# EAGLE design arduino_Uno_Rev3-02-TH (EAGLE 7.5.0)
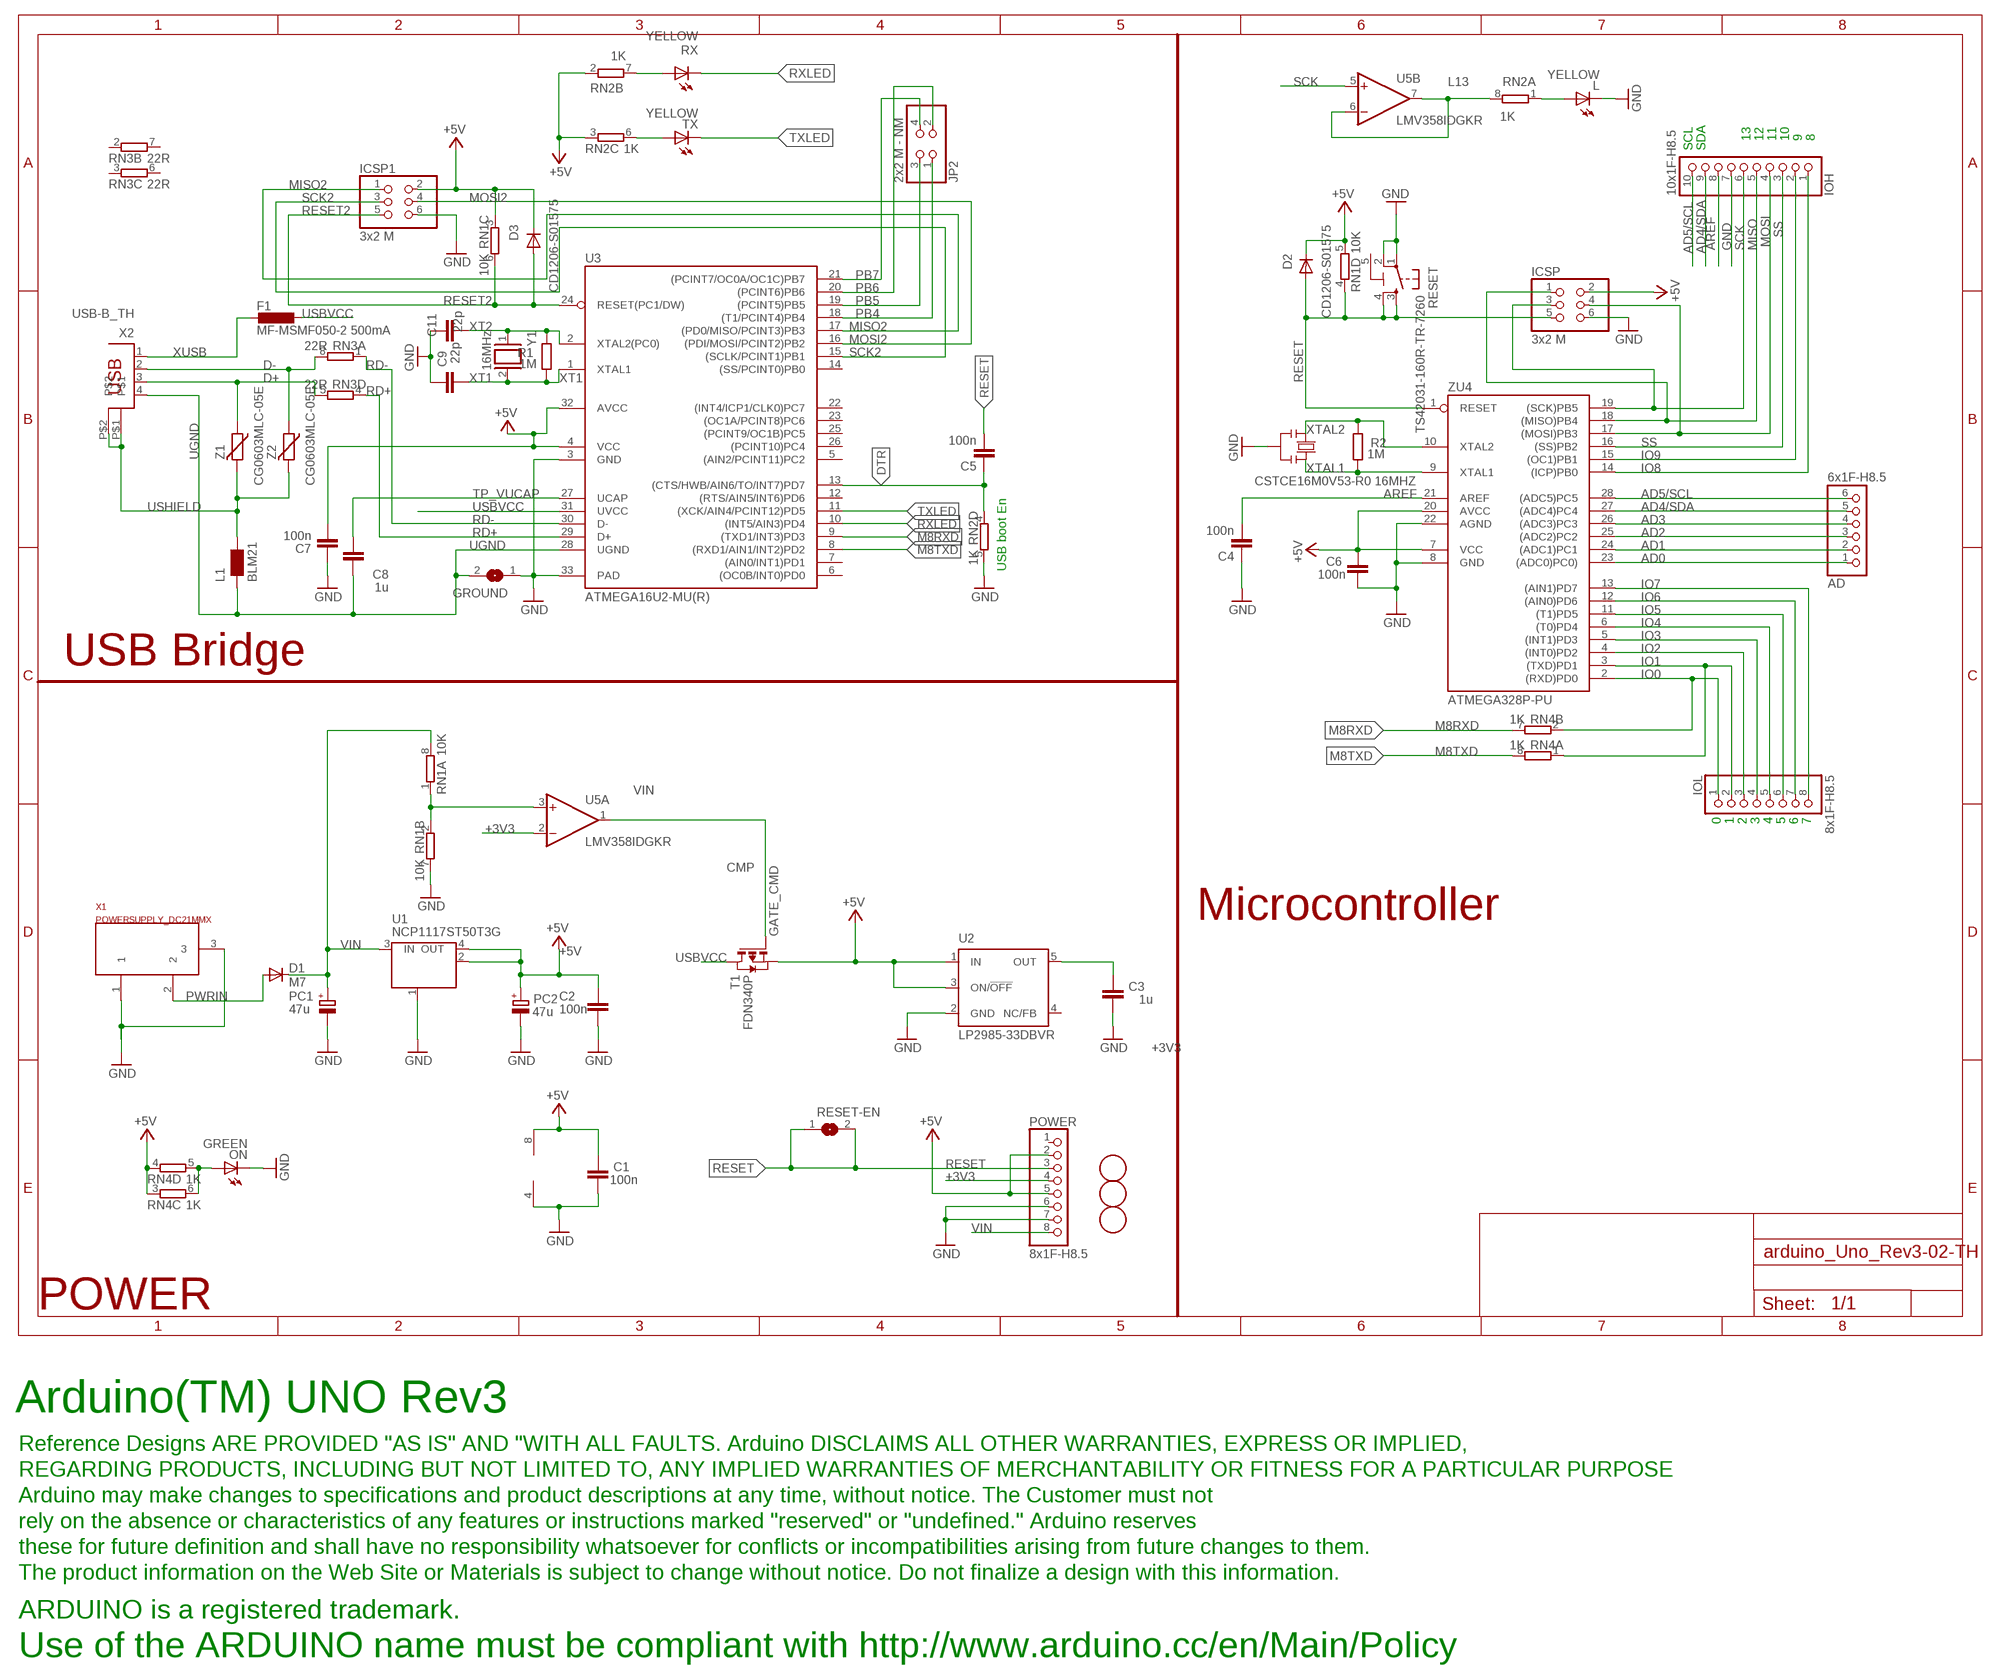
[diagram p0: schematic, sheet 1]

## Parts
AD  6x1F-H8.5  PINHD-1X6  [1X06]
C1  100n  C-EU0603-RND  [C0603-ROUND]
C2  100n  C-EU0603-RND  [C0603-ROUND]
C3  1u  C-EU0603-RND  [C0603-ROUND]
C4  100n  C-EU0603-RND  [C0603-ROUND]
C5  100n  C-EU0603-RND  [C0603-ROUND]
C6  100n  C-EU0603-RND  [C0603-ROUND]
C7  100n  C-EU0603-RND  [C0603-ROUND]
C8  1u  C-EU0603-RND  [C0603-ROUND]
C9  22p  C-EU0603-RND  [C0603-ROUND]
C11  22p  C-EU0603-RND  [C0603-ROUND]
D1  M7  DIODE-SMB  [SMB]
D2  CD1206-S01575  DIODE-MINIMELF  [MINIMELF]
D3  CD1206-S01575  DIODE-MINIMELF  [MINIMELF]
F1  MF-MSMF050-2 500mA  L-EUL1812  [L1812]
FD1  FIDUCIALMOUNT  [FIDUCIA-MOUNT]
FD2  FIDUCIALMOUNT  [FIDUCIA-MOUNT]
FD3  FIDUCIALMOUNT  [FIDUCIA-MOUNT]
GROUND  SJ  [SJ]
ICSP  3x2 M  PINHD-2X3  [2X03]
ICSP1  3x2 M  PINHD-2X3  [2X03]
IOH  10x1F-H8.5  PINHD-1X10_ARD  [1X10]
IOL  8x1F-H8.5  PINHD-1X8  [1X08]
JP2  2x2 M - NM  PINHD-2X2  [2X02]
L  YELLOW  LEDCHIP-LED0805  [CHIP-LED0805]
L1  BLM21  WE-CBF_0805  [0805]
ON  GREEN  LEDCHIP-LED0805  [CHIP-LED0805]
PC1  47u  CPOL-EUD  [PANASONIC_D]
PC2  47u  CPOL-EUD  [PANASONIC_D]
POWER  8x1F-H8.5  PINHD-1X8  [1X08]
R1  1M  R-EU_R0603  [R0603-ROUND]
R2  1M  R-EU_R0603  [R0603-ROUND]
RESET  TS42031-160R-TR-7260  TS42  [TS42]
RESET-EN  SJ  [SJ]
RN1  10K  4R-NCAY16  [CAY16]
RN2  1K  4R-NCAY16  [CAY16]
RN3  22R  4R-NCAY16  [CAY16]
RN4  1K  4R-NCAY16  [CAY16]
RX  YELLOW  LEDCHIP-LED0805  [CHIP-LED0805]
T1  FDN340P  PMOSSOT23  [SOT-23]
TX  YELLOW  LEDCHIP-LED0805  [CHIP-LED0805]
U1  NCP1117ST50T3G  MC33269ST-3.3T3  [SOT223]
U2  LP2985-33DBVR  LP2985-XXDBVR33  [SOT23-DBV]
U3  ATMEGA16U2-MU(R)  ATMEGA16U2-MU  [MLF32]
U5  LMV358IDGKR  LMV358MMX  [MSOP08]
U$1  DISCLAIMER  [DISCLAIMER]
X1  POWERSUPPLY_DC21MMX  [POWERSUPPLY_DC-21MM]
X2  USB-B_TH  PN61729  [PN61729]
Y1  16MHz  XTAL/S  [QS]
Y2  CSTCE16M0V53-R0 16MHZ  RESONATORMU  [RESONATOR]
Z1  CG0603MLC-05E  VARISTORCN0603  [CT/CN0603]
Z2  CG0603MLC-05E  VARISTORCN0603  [CT/CN0603]
ZU4  ATMEGA328P-PU  [DIL28-3]

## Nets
+3V3: C3.2 POWER.4 U2.5(OUT) U5.2(A:-IN)
+5V [usbvcc]: C1.2 C2.2 C6.2 C7.1 D2.C D3.C ICSP1.2 ICSP.2 PC2.+ POWER.2 POWER.5 RN1.3 RN1.5 RN2.2 RN2.3 RN4.3 RN4.4 T1.2(S) U1.2(OUT) U1.4(OUT) U2.1(IN) U2.3(ON/!OFF) U3.4(VCC) U3.32(AVCC) U5.8(P:V+) ZU4.7(VCC) ZU4.20(AVCC)
AD0: AD.1 ZU4.23((ADC0)PC0))
AD1: AD.2 ZU4.24((ADC1)PC1)
AD2: AD.3 ZU4.25((ADC2)PC2)
AD3: AD.4 ZU4.26((ADC3)PC3)
AD4/SDA: AD.5 IOH.9 ZU4.27((ADC4)PC4)
AD5/SCL: AD.6 IOH.10 ZU4.28((ADC5)PC5)
AREF [aref]: C4.2 IOH.8 ZU4.21(AREF)
CMP: RN1.1 RN1.2 U5.3(A:+IN)
D+: RN3.5 X2.3 Z1.1
D-: RN3.8 X2.2 Z2.1
DTR: C5.1 RN2.4 U3.13((CTS/HWB/AIN6/TO/INT7)PD7)
GATE_CMD: T1.3(G) U5.1(A:OUT)
GND [gnd]: C1.1 C2.1 C3.1 C4.1 C6.1 C7.2 C9.2 C11.2 GROUND.1 ICSP1.6 ICSP.6 IOH.7 L.C ON.C PC1.- PC2.- POWER.6 POWER.7 RESET.1 RESET.2 RN1.7 RN2.5 U1.1(GND/ADJ) U2.2(GND) U3.3(GND) U3.33(PAD) U5.4(P:V-) X1.1 X1.3 Y2.2 ZU4.8(GND) ZU4.22(AGND)
IO0: IOL.1 RN4.2 ZU4.2((RXD)PD0)
IO1: IOL.2 RN4.1 ZU4.3((TXD)PD1)
IO2: IOL.3 ZU4.4((INT0)PD2)
IO3: IOL.4 ZU4.5((INT1)PD3)
IO4: IOL.5 ZU4.6((T0)PD4)
IO5: IOL.6 ZU4.11((T1)PD5)
IO6: IOL.7 ZU4.12((AIN0)PD6)
IO7: IOL.8 ZU4.13((AIN1)PD7)
IO8: IOH.1 ZU4.14((ICP)PB0)
IO9: IOH.2 ZU4.15((OC1)PB1)
L13: RN2.8 U5.6(B:-IN) U5.7(B:OUT)
M8RXD: RN4.7 U3.9((TXD1/INT3)PD3)
M8TXD: RN4.8 U3.8((RXD1/AIN1/INT2)PD2)
MISO: ICSP.1 IOH.5 ZU4.18((MISO)PB4)
MISO2: ICSP1.1 U3.17((PD0/MISO/PCINT3)PB3)
MOSI: ICSP.4 IOH.4 ZU4.17((MOSI)PB3)
MOSI2: ICSP1.4 U3.16((PDI/MOSI/PCINT2)PB2)
N$1: L.A RN2.1
N$3: ON.A RN4.5 RN4.6
N$35: RN2.7 RX.A
N$36: RN2.6 TX.A
PB4: JP2.1 U3.18((T1/PCINT4)PB4)
PB5: JP2.3 U3.19((PCINT5)PB5)
PB6: JP2.2 U3.20((PCINT6)PB6)
PB7: JP2.4 U3.21((PCINT7/OC0A/OC1C)PB7)
PWRIN [power]: D1.A X1.2
RD+: RN3.4 U3.29(D+)
RD-: RN3.1 U3.30(D-)
RESET: C5.2 D2.A ICSP.5 POWER.3 RESET-EN.1 RESET-EN.2 RESET.3 RESET.4 RN1.4 ZU4.1(RESET)
RESET2: D3.A ICSP1.5 RN1.6 U3.24(RESET(PC1/DW))
RXLED: RX.C U3.10((INT5/AIN3)PD4)
SCK: ICSP.3 IOH.6 U5.5(B:+IN) ZU4.19((SCK)PB5)
SCK2: ICSP1.3 U3.15((SCLK/PCINT1)PB1)
SS: IOH.3 ZU4.16((SS)PB2)
TP_VUCAP: C8.1 U3.27(UCAP)
TXLED: TX.C U3.11((XCK/AIN4/PCINT12)PD5)
UGND [gnd]: C8.2 GROUND.2 L1.1 U3.28(UGND) X2.4
USBVCC [usbvcc]: F1.1 T1.1(D) U3.31(UVCC)
USHIELD [gnd]: L1.2 X2.P$1 X2.P$2 Z1.2 Z2.2
VIN [power]: D1.C PC1.+ POWER.8 RN1.8 U1.3(IN)
XT1: C9.1 R1.1 U3.1(XTAL1) Y1.2
XT2: C11.1 R1.2 U3.2(XTAL2(PC0)) Y1.1
XTAL1: R2.1 Y2.3 ZU4.9(XTAL1)
XTAL2: R2.2 Y2.1 ZU4.10(XTAL2)
XUSB [usbvcc]: F1.2 X2.1
Unconnected: POWER.1 RN3.2 RN3.3 RN3.6 RN3.7 U2.4(NC/FB) U3.5((AIN2/PCINT11)PC2) U3.6((OC0B/INT0)PD0) U3.7((AIN0/INT1)PD1) U3.12((RTS/AIN5/INT6)PD6) U3.14((SS/PCINT0)PB0) U3.22((INT4/ICP1/CLK0)PC7) U3.23((OC1A/PCINT8)PC6) U3.25((PCINT9/OC1B)PC5) U3.26((PCINT10)PC4)

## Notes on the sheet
- 13 | 12 | 11 | 10 | 9 | 8
- SCL | SDA
- USB boot En
- USB Bridge
- 0 | 1 | 2 | 3 | 4 | 5 | 6 | 7
- Microcontroller
- POWER
- Arduino(TM) UNO Rev3
- Use of the ARDUINO name must be compliant with http://www.arduino.cc/en/Main/Policy

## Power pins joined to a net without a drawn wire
5-GND: RESET.5(5-GND)

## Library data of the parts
AD = SmartPrj:PINHD-1X6: PIN HEADER
C1-C9 C11 = SmartPrj:C-EU: CAPACITOR, European symbol
D1-D3 = diode:DIODE-: DIODE
F1 = rcl:L-EU: INDUCTOR, European symbol
FD1-FD3 = SmartPrj:FIDUCIALMOUNT
GROUND RESET-EN = jumper:SJ: SMD solder JUMPER
ICSP ICSP1 = SmartPrj:PINHD-2X3: PIN HEADER
IOH = SmartPrj:PINHD-1X10_ARD: PIN HEADER
IOL POWER = SmartPrj:PINHD-1X8: PIN HEADER
JP2 = SmartPrj:PINHD-2X2: PIN HEADER
L ON RX TX = led:LED: LED
L1 = wuerth-elektronik:WE-CBF: SMD EMI Suppression Ferrite Beads
PC1 PC2 = rcl:CPOL-EU: POLARIZED CAPACITOR, European symbol
R1 R2 = SmartPrj:R-EU_: RESISTOR, European symbol
RESET = SmartPrj:TS42: TS42 Dongnan Electronics Tact switch VDC 12V - 50mA
RN1-RN4 = resistor-dil:4R-N: Array Chip Resistor Source: RS Component / Phycomp
T1 = zetex:PMOSSOT23: MOS FET
U1 = linear:MC33269ST*: Adjustable Output Low Dropout Voltage Regulator 800 mA Source: http://www.onsemi.com/pub/Collateral/MC33269-D.PDF
U2 = SmartPrj:LP2985-XXDBVR: ULTRALOW-POWER 50-mA LOW-DROPOUT LINEAR REGULATORS 50-mA Low-Dropout Regulator Source: http://focus.ti.com/lit/ds/symlink/tps77001.pdf
U3 = SmartPrj:ATMEGA16U2-
U5 = linear:LMV358?*: Dual General Purpose, Low Voltage, Rail-to-Rail Output Operational Amplifiers Source: http://www.national.com/mpf/LM/LMV321.html http://www.national.com/dt/lmv_qual.pdf
U$1 = SmartPrj:DISCLAIMER
X1 = SmartPrj:POWERSUPPLY_DC21MM
X2 = SmartPrj:PN61729: BERG USB connector
Y1 = SmartPrj:XTAL/S: CRYSTAL
Y2 = SmartPrj:RESONATOR
Z1 Z2 = varistor:VARISTOR: VARISTOR
ZU4 = SmartPrj:ATMEGA328P-: MICROCONTROLLER 4 Kbytes FLASH 128 bytes SRAM 256 bytes EEPROM UART 6-channel 10 bit ADC

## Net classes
0 default: width 0.254 mm, clearance 0.254 mm
1 power: width 0.61 mm, drill 0.61 mm, clearance 0.254 mm
2 gnd: width 0.305 mm, drill 0.559 mm, clearance 0.254 mm
3 usbvcc: width 0.508 mm, drill 0.61 mm, clearance 0.254 mm
4 aref: width 0.406 mm, drill 0.61 mm, clearance 0.254 mm

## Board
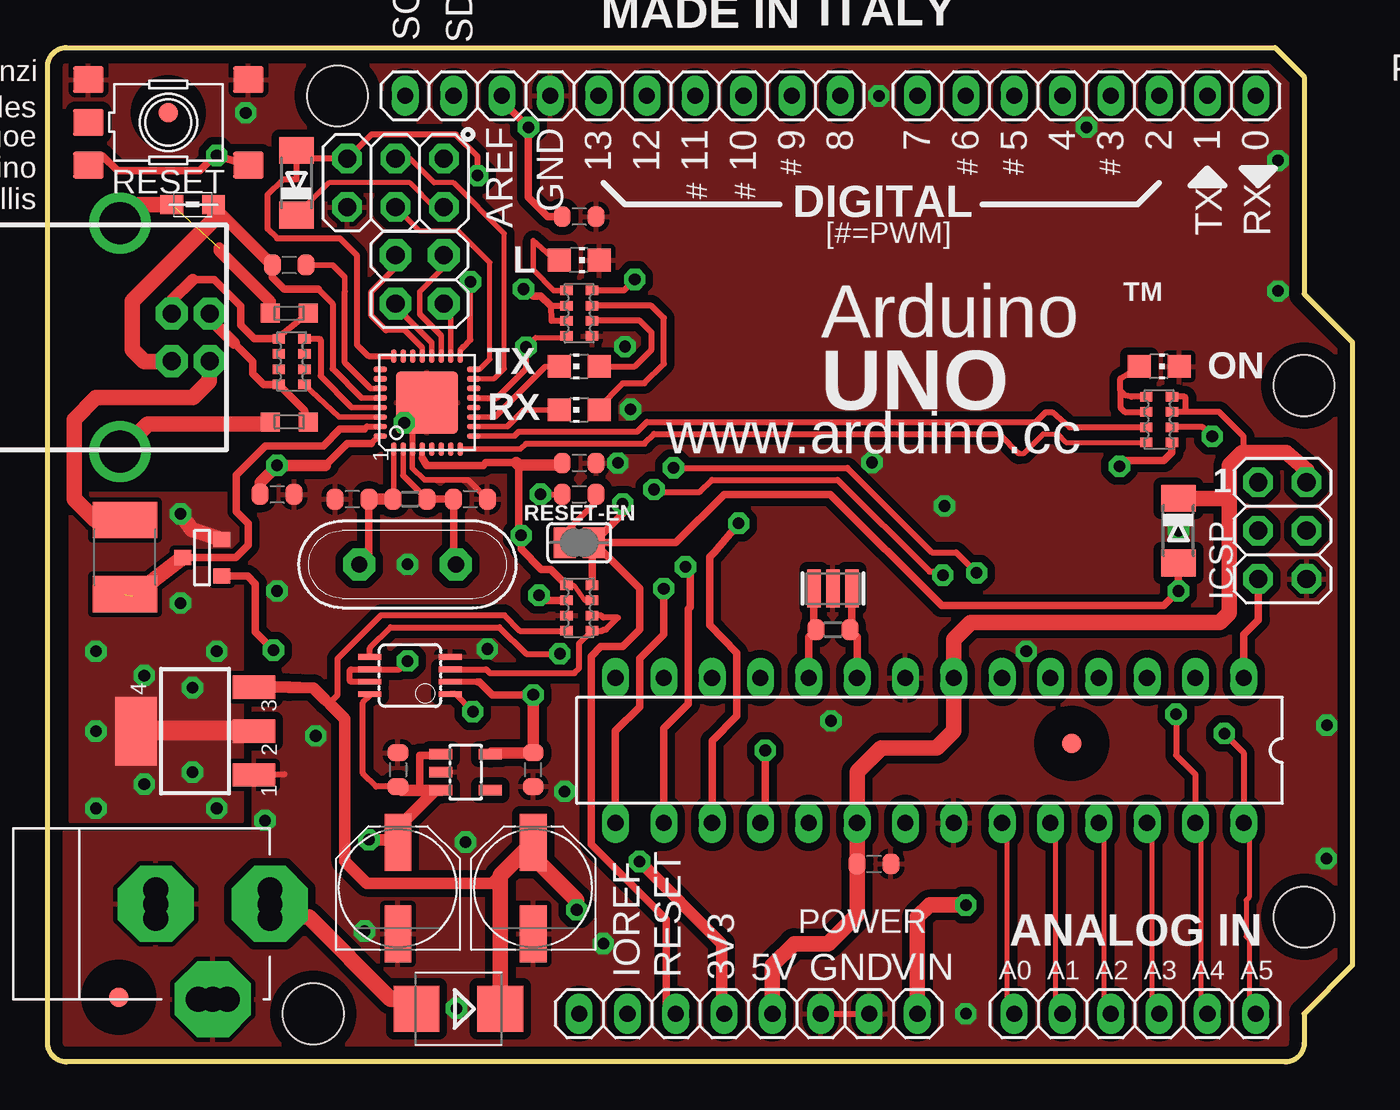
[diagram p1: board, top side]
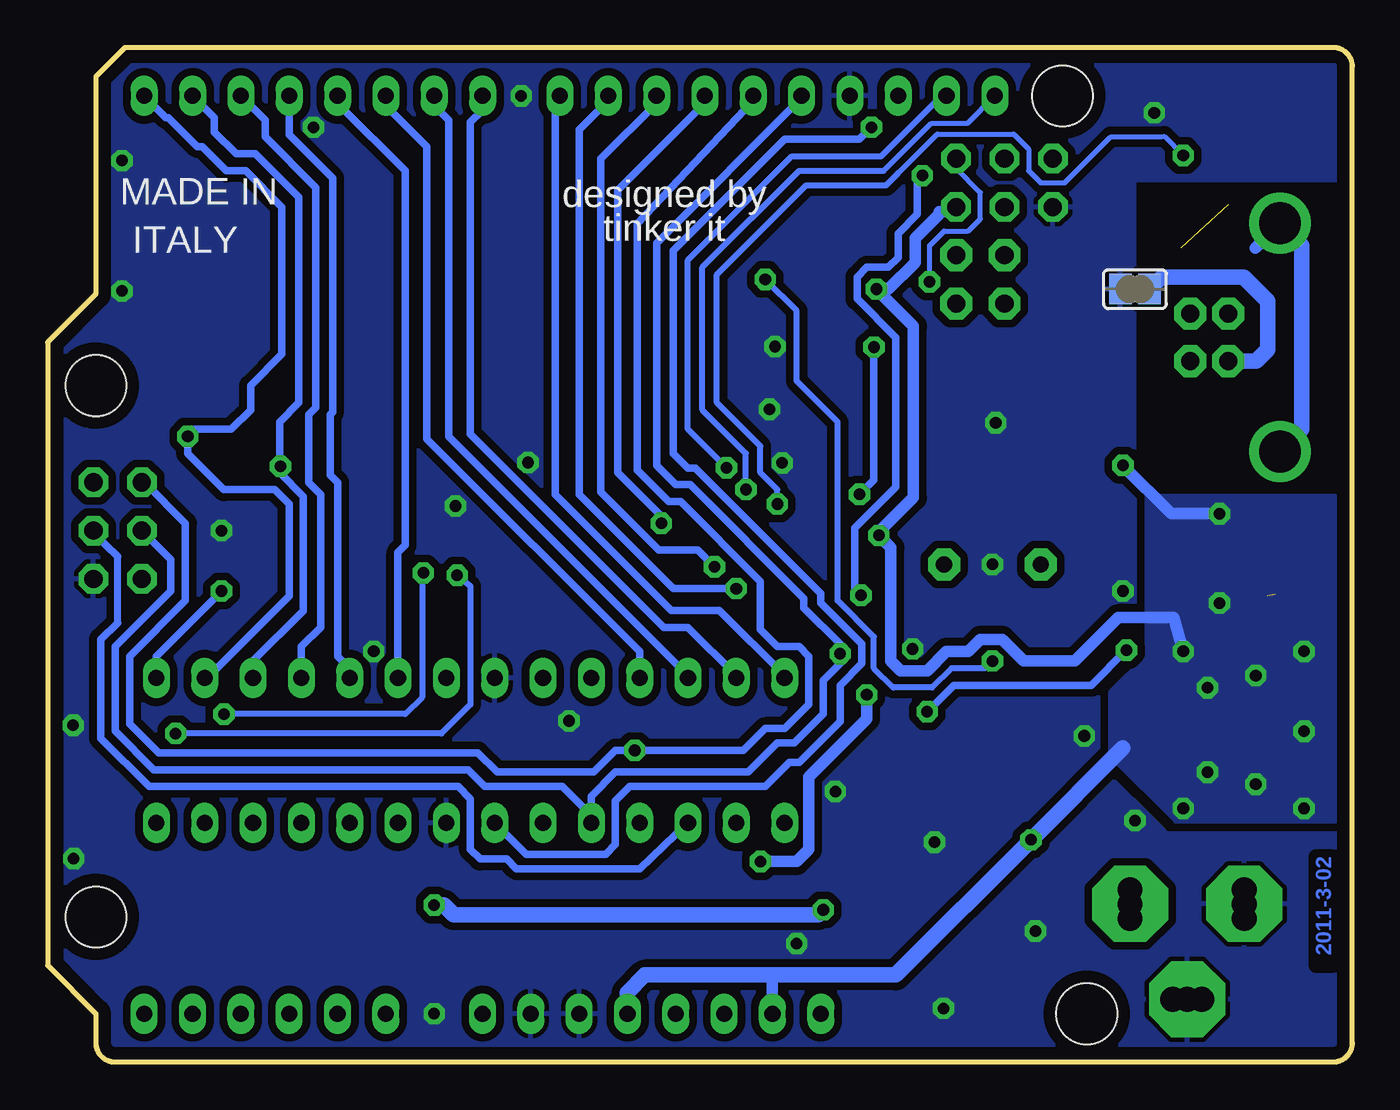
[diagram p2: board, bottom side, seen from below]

Size 68.58 x 53.34 mm. Coordinates in mm from the lower left corner, seen from the top.
Outline: 64.52,53.34 66.04,51.82 66.04,40.39 68.58,37.85 68.58,5.08 66.04,2.54 66.04,1 arc-90 65.04,0 1,0 arc-90 0,1 0,52.34 arc-90 1,53.34 64.52,53.34
Copper layers (1*16): Top 0.035mm / dielectric 1.5mm / Bottom 0.035mm
Design rules: minimum track width 10mil, minimum drill 22mil, track to track 10mil, track to pad 10mil, pad to pad 10mil, via to via 12mil, smd to smd 8mil, copper to edge 26mil, drill to drill 12mil, minimum pad ring 10mil, minimum via ring 10mil, stop-mask expansion 1mil, vias tented up to drill 30mil, thermal gap 10mil
Holes 3.2 mm at 66.04,35.56 66.04,7.62 15.24,50.8 13.97,2.54
vRestrict: area 22.9,44.1 to 24.6,49.1; area 25.4,45.5 to 27.1,49.1; area 28.4,45.3 to 29.6,48.8; area 31,45.3 to 32.1,48.8; area 33.5,45.3 to 34.7,48.8; area 36.1,45.3 to 37.2,48.8; area 38.7,47.2 to 39.9,48.8; area 40.3,45.1 to 47.6,46.9; area 60.3,44.2 to 61.7,46.7; area 62.9,44.2 to 64.3,46.7; area 61.3,35.8 to 64.8,37.2; area 0.6,21.8 to 2,30.1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

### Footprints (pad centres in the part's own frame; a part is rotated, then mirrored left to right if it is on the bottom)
1X06 = drill 0.85 pad 1.422 long: 1 -6.35,0; 2 -3.81,0; 3 -1.27,0; 4 1.27,0; 5 3.81,0; 6 6.35,0
C0603-ROUND = smd 0.898 x 1.1: 1 -0.889,0; 2 0.889,0
SMB = smd 2.4 x 2.4: A 2.2,0; C -2.2,0
MINIMELF = smd 1.4 x 1.8: A 1.7,0; C -1.7,0
L1812 = smd 1.9 x 3.4: 1 -1.95,0; 2 1.95,0
FIDUCIA-MOUNT = smd 1.016 x 1.016: P$1 0,0
SJ = smd 1.168 x 1.6: 1 -0.762,0; 2 0.762,0
2X03 = drill 0.95 pad 1.55 octagon: 1 -2.54,-1.27; 2 -2.54,1.27; 3 0,-1.27; 4 0,1.27; 5 2.54,-1.27; 6 2.54,1.27
1X10 = drill 0.85 pad 1.422 long: 1 -11.43,0; 2 -8.89,0; 3 -6.35,0; 4 -3.81,0; 5 -1.27,0; 6 1.27,0; 7 3.81,0; 8 6.35,0; 9 8.89,0; 10 11.43,0
1X08 = drill 0.85 pad 1.422 long: 1 -8.89,0; 2 -6.35,0; 3 -3.81,0; 4 -1.27,0; 5 1.27,0; 6 3.81,0; 7 6.35,0; 8 8.89,0
2X02 = drill 0.95 pad 1.676 octagon: 1 -1.27,-1.27; 2 -1.27,1.27; 3 1.27,-1.27; 4 1.27,1.27
CHIP-LED0805 = smd 1.2 x 1.2: A 0,-1.05; C 0,1.05
0805 = smd 1.2 x 1: 1 -1.1,0; 2 1.1,0
PANASONIC_D = smd 3 x 1.4: + 2.4,0; - -2.4,0
R0603-ROUND = smd 0.898 x 1.1: 1 -0.889,0; 2 0.889,0
TS42 = smd 1.6 x 1.4: 1 -4.2,2.25; 2 4.2,2.25; 3 -4.2,-2.25; 4 4.2,-2.25; 5 -4.2,0
CAY16 = smd 0.5 x 0.65: 1 -1.2,-0.675; 2 -0.4,-0.675; 3 0.4,-0.675; 4 1.2,-0.675; 5 1.2,0.675; 6 0.4,0.675; 7 -0.4,0.675; 8 -1.2,0.675
SOT-23 = smd 0.787 x 0.889: 1 0.025,-1.016; 2 -0.94,1.016; 3 0.991,1.016
SOT223 = smd 1.219 x 2.235: 1 -2.311,-3.099; 2 0,-3.099; 3 2.311,-3.099 | smd 3.6 x 2.2: 4 0,3.099
SOT23-DBV = smd 0.55 x 1.2: 1 -0.95,-1.3; 2 0,-1.3; 3 0.95,-1.3; 4 0.95,1.3; 5 -0.95,1.3
MLF32 = smd 0.7 x 0.28: 1 -2.45,1.75; 2 -2.45,1.25; 3 -2.45,0.75; 4 -2.45,0.25; 5 -2.45,-0.25; 6 -2.45,-0.75; 7 -2.45,-1.25; 8 -2.45,-1.75; 17 2.45,-1.75; 18 2.45,-1.25; 19 2.45,-0.75; 20 2.45,-0.25; 21 2.45,0.25; 22 2.45,0.75; 23 2.45,1.25; 24 2.45,1.75 | smd 0.28 x 0.7: 9 -1.75,-2.45; 10 -1.25,-2.45; 11 -0.75,-2.45; 12 -0.25,-2.45; 13 0.25,-2.45; 14 0.75,-2.45; 15 1.25,-2.45; 16 1.75,-2.45; 25 1.75,2.45; 26 1.25,2.45; 27 0.75,2.45; 28 0.25,2.45; 29 -0.25,2.45; 30 -0.75,2.45; 31 -1.25,2.45; 32 -1.75,2.45 | smd 3.254 x 3.254: 33 0,0
MSOP08 = smd 0.3 x 1.2: 1 -0.976,-2.113; 2 -0.326,-2.113; 3 0.324,-2.113; 4 0.974,-2.113; 5 0.974,2.112; 6 0.324,2.112; 7 -0.326,2.112; 8 -0.976,2.112
POWERSUPPLY_DC-21MM = drill 1.3 pad 4 octagon: 1 -5.08,-3.353; 2 -0.076,-6.35; 3 -0.076,-0.356 | drill 1.3: 4 -5.08,-4.115; 5 -5.08,-2.591; 6 -0.838,-0.356; 7 0.686,-0.356; 8 -0.838,-6.35; 9 0.686,-6.35
PN61729 = drill 0.95 pad 1.676 octagon: 1 1.25,4.71; 2 -1.25,4.71; 3 -1.25,2.71; 4 1.25,2.71 | drill 2.2: P$1 -6,0; P$2 6,0
QS = drill 0.85 pad 1.676 octagon: 1 -2.54,0; 2 2.54,0
RESONATOR = smd 0.7 x 2: 1 -1,0; 2 0,0; 3 1,0
CT/CN0603 = smd 1 x 1: 1 -1,0; 2 1,0
DIL28-3 = drill 0.85 pad 1.422 long: 1 -16.51,-3.81; 2 -13.97,-3.81; 3 -11.43,-3.81; 4 -8.89,-3.81; 5 -6.35,-3.81; 6 -3.81,-3.81; 7 -1.27,-3.81; 8 1.27,-3.81; 9 3.81,-3.81; 10 6.35,-3.81; 11 8.89,-3.81; 12 11.43,-3.81; 13 13.97,-3.81; 14 16.51,-3.81; 15 16.51,3.81; 16 13.97,3.81; 17 11.43,3.81; 18 8.89,3.81; 19 6.35,3.81; 20 3.81,3.81; 21 1.27,3.81; 22 -1.27,3.81; 23 -3.81,3.81; 24 -6.35,3.81; 25 -8.89,3.81; 26 -11.43,3.81; 27 -13.97,3.81; 28 -16.51,3.81

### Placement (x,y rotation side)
AD  57.15,2.54 0 top
C1  18.41,15.37 270 top
C2  12.06,29.84 180 top
C3  25.53,15.37 90 top
C4  27.94,44.45 180 top
C5  27.94,29.84 0 top
C6  43.43,10.41 180 top
C7  27.94,31.5 0 top
C8  12.7,41.91 180 top
C9  16,29.59 180 top
C11  22.23,29.59 0 top
D1  21.59,2.79 180 top
D2  59.44,27.94 270 top
D3  13.08,46.23 90 top
F1  4.06,26.54 90 top
FD1  6.35,49.91 0 top
FD2  53.84,16.74 0 top
FD3  3.73,3.41 0 top
GROUND  11.43,40.64 0 bottom
ICSP  64.9,27.94 270 top
ICSP1  18.29,46.23 180 top
IOH  30.23,50.8 180 top
IOL  54.61,50.8 180 top
JP2  19.56,41.15 90 top
L  27.94,42.16 270 top
L1  7.62,45.09 180 top
ON  58.42,36.58 270 top
PC1  25.53,9.14 90 top
PC2  18.41,9.14 90 top
POWER  36.83,2.54 0 top
R1  19.05,29.59 0 top
R2  41.27,22.73 180 top
RESET  6.35,49.4 0 top
RESET-EN  27.94,27.3 0 top
RN1  27.94,23.88 90 top
RN2  27.94,39.37 270 top
RN3  12.83,36.83 90 top
RN4  58.42,33.78 90 top
RX  27.94,34.29 90 top
T1  8.13,26.54 270 top
TX  27.94,36.58 90 top
U1  7.75,17.4 90 top
U2  21.97,15.24 270 top
U3  19.94,34.67 90 top
U5  19.05,20.32 90 top
U$1  not placed on the board
X1  5.33,8.38 90 top
X2  3.81,38.1 270 top
Y1  18.92,26.16 180 top
Y2  41.27,24.89 0 top
Z1  12.7,39.37 180 top
Z2  12.7,33.66 180 top
ZU4  46.35,16.38 180 top

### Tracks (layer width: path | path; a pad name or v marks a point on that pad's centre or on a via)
+3V3  (via drill 0.61)
  Top 0.305: 22.61,19.99 U5.2
  Top 0.406: 22.61,19.99 22.68,19.99 23.37,19.3 v25.53,19.3
  Top 0.61: v31.11,10.54 35.43,6.22 35.43,2.67 POWER.4 | U2.5 23.34,16.26 C3.2 v25.53,19.3
  Bottom 0.61: v31.11,10.54 29.21,10.54 28.57,11.18 28.57,14.99 25.53,18.03 v25.53,19.3
+5V  (via drill 0.61)
  Top 0.254: 27.32,25.02 RN1.5 27.65,25.08 28.23,24.28 RN1.3 | ICSP1.2 20.32,44.96 19.05,46.23 14.78,46.23 D3.C
  Top 0.305: 59.82,34.18 61.58,34.18 62.87,32.89 62.87,32.05 | 59.82,34.18 RN4.3 | RN4.4 59.76,34.98 59.82,34.92 59.82,34.18 | RN2.2 26.43,39.77 26.47,38.97 RN2.3 | 19.69,31.75 U3.4 | U3.32 17.43,32.92 17.02,32.51 | U5.8 16.98,19.3 16.57,18.9 16.57,15.18 17.27,14.48 C1.2
  Top 0.406: 42.55,10.16 42.35,10.35 | 26.43,39.77 25.93,40.28 25.53,40.26 v25.02,40.64 | RN1.5 26.43,25.91 25.96,25.91 24.89,26.97 v24.89,27.69 24.77,28.19 24.77,31.38 | 24.64,31.51 23.03,31.51 22.89,31.37 19.94,31.37 19.69,31.75 | 17.02,32.51 15.75,32.51 14.61,31.37 | U2.1 20.61,16.13 19.56,16.13 19.56,14.29
  Top 0.508: 11.02,17.42 U1.2 | ICSP.2 66.04,30.48
  Top 0.61: C6.2 42.58,10.88 42.55,11.43 | 24.64,31.51 24.77,31.38 26.94,31.38 C7.1 | 11.05,29.72 C2.2 11.18,30.48 v12.06,31.37 14.61,31.37 | v16.89,11.68 18.78,11.68 PC2.+ 18.41,12.32 20.39,14.29 U2.3 19.56,14.29 18.6,14.29 C1.2
  Top 0.813: 66.17,30.44 ICSP.2 66.17,31.11 65.1,32.05 62.87,32.05 62.79,32.05 62.1,31.37 62.1,29.46 | 62.1,29.46 62.1,23.62 61.59,23.11 48.51,23.11 47.62,22.23 ZU4.7 47.62,17.4 46.74,16.51 43.81,16.51 42.55,15.24 ZU4.20 42.55,11.43 C6.2 42.55,10.16 42.55,7.75 41.02,6.22 39.24,6.22 38.1,5.08 POWER.5 | T1.2 7.57,27.99 v6.99,28.83 | D2.C 61.93,29.64 62.1,29.46
  Top 1.016: U1.4 5.84,17.4 5.87,17.42 11.02,17.42
  Bottom 0.61: ICSP1.2 21.08,44.7 21.72,44.7 21.72,44.58 22.99,43.31 22.99,42.04 24.38,40.64 v25.02,40.64 23.07,38.69 23.07,29.68 24.89,27.85 v24.89,27.69 24.26,27.05 24.26,21.08 23.75,20.57 22.35,20.57 21.34,21.59 20.19,21.59 19.56,22.23 18.41,22.23 17.27,21.08 14.61,21.08 12.32,23.37 9.4,23.37 v8.89,21.59 | POWER.2 30.48,4.7 30.61,4.57 | v12.06,31.37 9.53,28.83 v6.99,28.83
  Bottom 0.813: POWER.5 38.12,3.63 37.19,4.57 30.61,4.57 24,4.57 v16.89,11.68 12.06,16.51
  other vias: 2.54,21.59 5.08,20.32 6.99,24.13 2.54,13.34 5.08,14.61 2.54,17.4 8.89,13.34 7.62,15.24 7.62,19.68
  pour Bottom (isolate 0.406, no thermals): 0.89,29.72 10.79,29.72 10.79,21.34 12.7,19.43 12.7,16.13 9.27,12.7 0.89,12.7
  pour Top (no thermals): 1.27,12.7 1.27,29.84 10.16,29.84 10.16,12.7
AD0
  Top 0.254: ZU4.23 50.44,12.17 50.44,3 AD.1
AD1
  Top 0.254: ZU4.24 52.98,12.17 52.98,3 AD.2
AD2
  Top 0.254: ZU4.25 55.52,12.17 55.52,3 AD.3
AD3
  Top 0.254: ZU4.26 58.06,12.17 58.06,3 AD.4
AD4/SDA  (via drill 0.61)
  Top 0.254: ZU4.27 60.6,12.17 60.6,3 AD.5
  Top 0.305: v32.89,31.24 42.04,31.24 46.48,26.8 47.75,26.8 v48.83,25.72 49.02,25.65 | v59.31,18.29 59.31,16.13 60.33,15.11 ZU4.27
  Bottom 0.305: IOH.9 21.59,50.8 24.77,47.62 29.46,47.62 34.92,42.16 34.92,33.27 v32.89,31.24 | v48.83,25.72 48.9,25.65 48.9,19.18 49.78,18.29 v59.31,18.29
AD5/SCL  (via drill 0.61)
  Top 0.254: ZU4.28 63.14,12.17 63.14,8.66 62.99,8.51 62.99,6.6 63.14,6.45 63.14,3 AD.6
  Top 0.305: v31.88,30.1 31.88,29.97 34.29,29.97 34.92,30.61 41.53,30.61 46.35,25.78 46.86,25.78 v47.05,25.59 | ZU4.28 62.87,16.26 v61.85,17.27
  Bottom 0.254: IOH.10 20.22,49.35 22.12,49.35 24.64,46.86
  Bottom 0.305: v61.85,17.27 47.88,17.27 46.35,18.8 46.35,25.02 v47.05,25.59 | v31.88,30.1 31.88,32 34.16,34.29 34.16,41.78 29.08,46.86 24.64,46.86
AREF  (via drill 0.61)
  Top 0.406: IOH.8 23.88,50.55 v25.27,49.15 25.27,45.47 26.29,44.45 C4.2
  Bottom 0.406: ZU4.21 43.43,10.92 39.24,10.92 38.73,11.43 38.73,13.72 37.97,14.48 30.86,14.48 29.59,15.75 29.08,15.75 26.92,17.91 26.92,19.81 25.78,20.95 25.78,21.97 27.94,24.13 27.94,24.64 34.54,31.24 34.92,31.24 35.69,32 35.69,42.67 29.84,48.51 25.91,48.51 v25.27,49.15
CMP
  Top 0.305: U5.3 23.04,20.64 23.24,20.45 27.69,20.45 27.94,20.7 27.94,22 RN1.1 29.15,22.68 29.21,22.73 29.34,22.73 29.97,23.37 29.21,23.37 29.1,23.48 RN1.2
D+
  Top 0.305: Z1.1 12.1,38.1 RN3.5
  Top 0.406: 7.62,41.15 8.76,41.15 10.16,39.75 10.16,38.73 10.87,38.03 RN3.5
  Top 0.61: X2.3 6.52,40.05 7.62,41.15
  Bottom 0.61: X2.3 6.5,39.37
D-
  Top 0.406: 9.82,37.81 10.79,36.83 10.79,36.2 11.36,35.63 RN3.8 13.49,34.29 Z2.1
  Top 0.61: X2.2 8.53,39.1 9.82,37.81
  Bottom 0.305: X2.2
DTR  (via drill 0.61)
  Top 0.254: v25.15,37.59 25.65,38.1 27.2,38.1
  Top 0.305: 26.42,29.84 C5.1 | 27.2,38.1 RN2.4 | U3.13 23.62,34.92 25.15,36.45 v25.15,37.59
  Top 0.406: v25.91,29.84 26.42,29.84
  Bottom 0.406: v25.15,37.59 25.15,30.61 v25.91,29.84
GATE_CMD  (via drill 0.61)
  Top 0.305: U5.1 21.42,19.34 v22.35,18.41
  Top 0.406: T1.3 10.52,25.55 10.92,25.15 10.92,22.61 11.62,21.91 v11.87,21.65 12.06,21.46
  Bottom 0.406: v22.35,18.41 20.95,19.81 13.72,19.81 v11.87,21.65
GND  (via drill 0.61)
  Top 0.279: C11.2 22.1,30.61 19.81,30.61 19.18,31.24 19.18,32.26
  Top 0.305: POWER.6 POWER.7 | U1.1 12.45,15.14 | U3.3 19.19,33.52 v18.75,33.6 U3.33
  Bottom 0.305: GROUND.1 10.79,40.64
  other vias: 29.21,6.22 27.18,14.22 16.66,6.88 30.63,34.32 54.61,49.15 30.35,37.62 11.43,12.7 41.17,17.93 51.44,21.59 29.97,31.5 43.69,50.8 48.26,2.54 59.44,27.94 21.49,2.82 67.21,10.69 64.67,47.4 12.06,24.77 67.23,17.7 23.11,21.72 10.41,49.91 47.14,29.24 18.92,26.16 43.33,31.52 21.97,11.56 14.1,17.14 64.67,40.54
  pour Bottom (isolate 0.406, rank 2): 0.64,52.7 67.69,52.7 67.94,52.45 67.94,0.64 0.89,0.64 0.64,0.89 0.64,30.1 11.43,30.1 11.43,46.35 0.64,46.35
  pour Top (isolate 0.406, rank 2): 0.64,52.7 67.94,52.7 67.94,0.64 0.64,0.64 0.51,30.48 11.43,30.48 11.43,46.35 0.64,46.35
IO0  (via drill 0.61)
  Top 0.305: RN4.2 60.73,33.38 v61.21,32.89
  Bottom 0.406: ZU4.2 60.2,20.19 55.88,24.51 55.88,29.34 56.64,30.1 59.31,30.1 61.21,32 v61.21,32.89 60.83,33.27 58.93,33.27 57.91,34.29 57.91,35.56 56.26,37.21 56.26,44.96 58.17,46.86 59.18,46.86 60.45,48.13 60.71,48.13 62.23,49.66 62.36,49.66 IOL.1
IO1  (via drill 0.61)
  Top 0.406: RN4.1 59.09,32.04 58.67,31.62 56.64,31.62 v56.34,31.32
  Bottom 0.406: ZU4.3 57.78,21.08 55.14,23.72 55.14,29.74 56.39,30.99 56.39,31.11 v56.34,31.32 56.39,31.37 56.39,33.66 55.37,34.67 55.37,45.47 57.66,47.75 58.67,47.75 59.82,48.9 59.82,49.66 IOL.2
IO2
  Bottom 0.406: ZU4.4 55.24,21.84 54.23,22.86 54.23,29.84 54.86,30.48 54.86,34.04 54.48,34.42 54.48,45.97 57.15,48.64 57.15,49.53 IOL.3
IO3
  Bottom 0.406: ZU4.5 52.7,20.7 53.34,21.34 53.34,30.48 53.72,30.86 53.72,34.04 53.59,34.16 53.59,46.48 55.88,48.77 IOL.4
IO4
  Bottom 0.406: IOL.5 53.21,50.29 49.78,46.86 49.78,27.18 50.16,26.8 ZU4.6
IO5
  Bottom 0.406: IOL.6 50.8,50.29 48.64,48.13 48.64,32.77 37.47,21.59 ZU4.11
IO6
  Bottom 0.406: IOL.7 48.26,50.29 47.5,49.53 47.5,32.89 34.92,20.32 ZU4.12
IO7
  Bottom 0.406: IOL.8 45.72,50.04 46.35,49.4 46.35,33.02 36.2,22.86 34.92,22.86 32.38,20.32 ZU4.13
IO8
  Bottom 0.406: ZU4.14 29.84,20.32 33.27,23.75 35.81,23.75 41.91,29.84 41.91,50.55 41.66,50.29 IOH.1
IO9  (via drill 0.61)
  Top 0.406: ZU4.15 29.84,17.4 31.11,18.67 31.11,21.21 32.38,22.48 v32.38,24.89
  Bottom 0.406: v32.38,24.89 35.69,24.89 40.64,29.84 40.64,49.02 39.12,50.55 IOH.2
L13  (via drill 0.61)
  Top 0.305: U5.7 15.95,19.99 15.88,20.07 15.88,20.57 15.95,20.64 U5.6 18.48,20.64 18.54,20.7 v18.92,21.08 | RN2.8 30.28,40.57 v30.86,41.15
  Bottom 0.305: v30.86,41.15 29.21,39.5 29.21,35.81 27.05,33.66 27.05,24.26 25.15,22.35 25.15,20.7 24.13,19.68 22.1,19.68 21.08,20.7 19.3,20.7 v18.92,21.08
M8RXD
  Top 0.279: U3.9 24.54,32.92 24.77,33.15
  Top 0.305: RN4.7 53.7,33.38 52.79,34.16 52.45,34.16 51.94,33.66 31.5,33.66 30.99,33.15 24.77,33.15
M8TXD
  Top 0.254: RN4.8 53.52,32.58 53.09,33.02 52.32,33.02 51.31,32 51.05,32
  Top 0.279: U3.8 24.86,32.22 25.15,32.51
  Top 0.305: 25.15,32.51 31.37,32.51 31.88,33.02 50.04,33.02 51.05,32
MISO  (via drill 0.61)
  Top 0.406: v37.72,16.38 37.72,12.83 ZU4.18
  Bottom 0.406: IOH.5 31.5,50.55 37.59,44.07 37.59,31.11 35.94,29.46 35.31,29.46 31.11,25.27 31.11,22.73 30.23,21.84 29.08,21.84 28.57,21.34 28.57,18.8 29.84,17.53 30.86,17.53 32,16.38 v37.72,16.38 | ICSP.1 63.45,30.43 61.34,28.32 61.34,24.26 64.26,21.34 64.26,17.78 62.74,16.26 45.97,16.26 44.96,15.24 39.88,15.24 38.73,16.38 v37.72,16.38 | v37.72,16.38 37.85,16.13 37.85,16.26
MISO2  (via drill 0.61)
  Top 0.254: v22.23,41.02 22.23,39.5
  Top 0.279: 21.84,37.59 21.69,37.44 U3.17
  Top 0.305: v22.23,41.02 22.23,37.97 21.84,37.59
  Bottom 0.254: v22.23,41.02 22.23,42.93 21.46,43.69 20.19,43.69 19.56,44.32 19.56,45.72 20.83,46.99 ICSP1.1
MOSI  (via drill 0.61)
  Top 0.406: ZU4.17 34.92,16.89 36.22,18.19 36.22,21.51 34.8,22.99 34.8,26.54 35.05,26.8 v36.32,28.32
  Bottom 0.381: 64.9,23.09 64.9,26.57
  Bottom 0.406: IOH.4 34.04,50.42 38.61,45.85 38.61,30.99 36.32,28.7 v36.32,28.32 | ICSP.4 66.18,27.83 64.9,26.57 | 64.9,23.09 65.79,22.23 65.79,17.02 63.25,14.48 46.99,14.48 46.35,13.84 46.35,11.18 45.85,10.67 44.45,10.67 43.94,10.16 37.47,10.16 ZU4.17
MOSI2
  Top 0.254: ICSP1.4 19.56,43.69 21.59,43.69 23.24,42.04 23.24,36.96 22.7,36.42 U3.16
N$1
  Top 0.279: RN2.1 26.61,40.57 25.53,41.66 25.53,43.18 26.67,42.16 L.A
N$3
  Top 0.305: RN4.6 56.62,34.18 56.39,34.42 56.39,35.31 | 56.39,35.31 56.39,35.94 ON.A | RN4.5 56.97,34.98 56.64,35.05 56.39,35.31
N$35
  Top 0.305: RX.A 28.96,34.29 28.96,34.42 30.23,35.69 31.37,35.69 32.38,36.7 32.38,39.12 31.73,39.77 RN2.7
N$36
  Top 0.305: TX.A 29.25,36.57 30.86,36.57 31.75,37.47 31.75,38.35 31.37,38.73 31.13,38.97 RN2.6
PB4
  Top 0.279: U3.18 21.19,39.52
  Top 0.305: 21.19,39.52 JP2.1
PB5
  Top 0.279: 20.83,41.78 19.56,40.51 19.56,39.32 20.69,38.19 U3.19
  Top 0.305: 20.83,41.78 JP2.3
PB6
  Top 0.279: U3.20 20.19,37.83 18.29,39.73 JP2.2
PB7
  Top 0.279: 17.78,38.48 18.77,38.48 19.69,37.56 U3.21
  Top 0.305: JP2.4 18.29,41.78 17.02,40.51 17.02,39.24 17.78,38.48
PWRIN
  Top 0.813: D1.A 18.88,3.3 18.03,3.3 13.72,7.62 12.37,7.62 X1.2
  Bottom 0.813: X1.2 11.73,8.26
RD+
  Top 0.279: U3.29 16,34.42 14.35,36.07
  Top 0.305: 14.35,36.07 14.35,37.97 14.29,38.03 RN3.4
RD-
  Top 0.254: RN3.1 13.53,35.63
  Top 0.279: U3.30 15.34,33.92 RN3.1
RESET  (via drill 0.61)
  Top 0.305: C5.2 28.83,29.46 27.18,27.81 RESET-EN.1
  Top 0.406: RESET-EN.2 RESET-EN.1 | ICSP.5 63.64,23.25 62.87,22.48 ZU4.1 | POWER.3 32.51,3.05 32.51,7.49 28.57,11.43 28.57,21.34 29.08,21.84 30.23,21.84 31.11,22.73 31.11,24.89 RESET-EN.2 | RN1.4 28.61,27.85 RESET-EN.2 | RESET.3 2.88,47.66 3.68,46.86 8,46.86 8.76,47.62 v8.89,47.66 RESET.4 | RESET-EN.2 33.02,27.3 35.56,29.84 41.15,29.84 46.99,24 58.67,24 v59.44,24.77 D2.A | v30.23,29.34 30.23,28.83 RESET-EN.2
  Bottom 0.254: v8.89,47.66 9.89,48.67 10.05,48.64 12.7,48.64 15.11,46.23 16.38,46.23 17.02,46.86 17.02,48.01 17.8,48.79 21.82,48.79 23.88,46.74
  Bottom 0.305: 23.88,46.74 24.51,46.1 28.7,46.1 33.4,41.4 33.4,34.67 31.11,32.38 31.11,30.99 30.23,30.1 v30.23,29.34
  Bottom 0.406: v59.44,24.77 62.87,21.34 ZU4.1
RESET2  (via drill 0.61)
  Top 0.305: v22.61,46.61 22.61,47.62 21.46,48.77 17.02,48.77 ICSP1.5 13.51,47.5 D3.A 13.08,46.4 12.37,46.4 11.56,45.59 11.56,45.39 11.56,43.81 12.06,43.31 15.37,43.31 16.26,42.42 16.26,37.72 16.85,37.12 U3.24
  Top 0.406: RN1.6 26.18,24.28 26.16,24.26 v25.84,24.53 v25.83,24.54
  Bottom 0.406: v22.61,46.61 22.86,46.35 22.86,44.58 23.88,43.56 23.88,42.29 24.38,41.78 25.53,41.78 26.04,41.27 26.04,40.13 24,38.1 24,30.23 26.16,28.07 26.16,24.87 v25.83,24.54
RXLED
  Top 0.279: RX.C 25.02,34.29 24.15,33.42 U3.10
SCK  (via drill 0.61)
  Top 0.305: v26.92,21.46 25.15,21.46 23.75,22.86 18.03,22.86 16.94,21.76 U5.5
  Bottom 0.406: ICSP.3 62.1,26.42 62.1,24.77 65.02,21.84 65.02,17.4 62.99,15.37 46.48,15.37 45.59,14.48 41.53,14.48 40.01,12.95 | 40.01,12.95 40.01,13.97 38.73,15.24 31.75,15.24 30.23,16.76 29.34,16.76 27.81,18.29 27.81,20.07 26.92,20.95 v26.92,21.46 26.92,21.97 28.83,23.88 28.83,24.38 34.8,30.35 35.56,30.35 36.58,31.37 36.58,43.05 28.96,50.67 IOH.6 | 40.01,12.95 ZU4.19
SCK2
  Top 0.254: U3.15 23.48,35.92 24,36.45 24,43.56 21.34,46.23 20.32,46.23 19.05,47.5 ICSP1.3
SS  (via drill 0.61)
  Top 0.406: v33.53,26.04 33.78,25.78 33.78,23.93 33.68,23.82 33.68,18.82 32.38,17.53 ZU4.16
  Bottom 0.406: v33.53,26.04 34.42,26.92 36.45,26.92 39.5,29.97 39.5,47.5 36.58,50.42 IOH.3
TP_VUCAP
  Top 0.279: U3.27 16.98,35.42 15.62,36.78 | 15.62,40.51 15.62,41.27 14.99,41.91 C8.1
  Top 0.305: 15.62,36.78 15.62,40.51
TXLED
  Top 0.279: U3.11 23.51,33.92 26.16,36.58 TX.C
UGND
  Top 0.279: U3.28 16.51,34.92 14.99,36.45
  Top 0.305: 14.99,36.45 14.99,39.88 14.22,40.64
  Top 0.406: C8.2 11.81,41.27 12.45,40.64 14.22,40.64
  Top 0.61: L1.1 8.72,45 C8.2
  Top 0.813: L1.1 8.85,44.41 4.45,40.01 4.45,37.47 5.08,36.83 6.5,36.83 X2.4
  Bottom 0.61: X2.4 6.5,36.83
  Bottom 0.813: X2.4 5.06,36.85 4.45,37.47 4.45,40.01 5.71,41.27 10.03,41.27 GROUND.2
USBVCC  (1 unrouted)
  Top 0.305: U3.31 16.78,33.42 16.64,33.27
  Top 0.406: 16.64,33.27 15.37,33.27 14.48,32.38 11.43,32.38 9.91,30.86 9.91,28.96 10.54,28.32 10.54,27.18 9.88,26.52 T1.1
  Top 0.813: 3.47,24.51 4.47,24.51 T1.1
USHIELD  (1 unrouted)
  Top 0.61: 9.02,42.8 9.02,42.67 11.7,39.99 Z1.2 | 11.06,33.54 11.19,33.54 11.3,33.66 Z2.2
  Top 0.813: L1.2 4.79,45.09 X2.P$1 | 11.06,33.54 5.25,33.54 X2.P$2
  Bottom 0.61: X2.P$1 5.11,42.8
  Bottom 0.813: X2.P$1 3.81,44.07 2.67,42.93 2.67,33.27 3.81,32.13 X2.P$2
VIN  (via drill 0.61)
  Top 0.305: RN1.8 24.82,22.68 24,23.5 17.53,23.5 15.24,21.21 15.24,19.3 14.8,18.86
  Top 0.61: 13.97,19.68 12.7,19.68 | 13.97,19.68 14.61,19.05 14.8,18.86 15.62,18.03 15.62,10.54 16.76,9.4 23.38,9.4 23.95,9.96 | 13.97,19.68 12.67,19.71 U1.3 | PC1.+ 25.54,11.43
  Top 0.813: v48.26,8.26 46.35,8.26 45.72,7.62 POWER.8 | D1.C 23.79,9.81 23.95,9.96 PC1.+ 25.53,10.79 27.81,8.51 v27.81,8
  Bottom 0.813: v48.26,8.26 47.75,8.26 47.24,7.75 28.07,7.75 v27.81,8
XT1
  Top 0.254: R1.1 18.29,29.72
  Top 0.279: 18.19,29.75 U3.1
  Top 0.305: R1.1 18.19,29.75
  Top 0.406: C9.1 16.89,26.67 16.51,26.67 Y1.2
  Top 0.61: C9.1 R1.1
XT2
  Top 0.279: 18.69,30.84 U3.2
  Top 0.305: R1.2 18.69,30.84
  Top 0.406: R1.2 C11.1 21.34,26.8 21.46,26.67 Y1.1
XTAL1
  Top 0.406: ZU4.9 42.55,22.35 R2.1 42.27,22.84 Y2.3
XTAL2
  Top 0.406: ZU4.10 40.01,22.35 R2.2 40.27,22.84 Y2.1
XUSB
  Top 0.813: F1.2 2.5,28.49 1.4,29.59 1.4,33.78 2.54,34.92 7.62,34.92 8.51,35.81 X2.1
  Bottom 0.305: X2.1 8.51,36.84

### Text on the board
Top: Use of the Arduino name must be compliant with http://www.arduino.cc/en/Main/Policy
Bottom: 2011-3-02
tPlace: MADE IN | ITALY | Prototype | Edition | Limited | 13 | 12 | 11 | 10 | 9 | 8 | 7 | 6 | 5 | 4 | 3 | 2 | 1 | 0
tNames: SCL | SDA | M.Banzi | D.Cuartielles | T.Igoe | AREF | GND | G.Martino | # | # | # | # | D.Mellis | # | # | DIGITAL | [#=PWM] | TX | RX | TM | TX | Arduino | RX | UNO | www.arduino.cc | 1 | ANALOG IN | IOREF | RESET | 3V3 | 5V | GND | VIN | A0 | A1 | A2 | A3 | A4 | A5
bNames: MADE IN | designed by | MADE IN | ITALY | tinker it | ITALY | designed by | tinker it | ATMEGA328
ReferenceLC: L | TX | ON | RX | PC1 | PC2
214bmp: D:/SmartProjects/Snc/a4_bn_logo2.bmp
